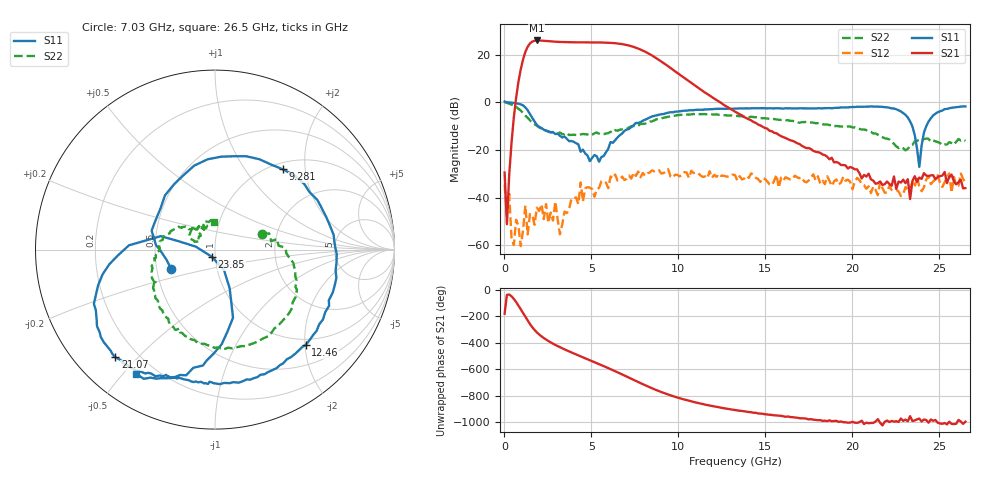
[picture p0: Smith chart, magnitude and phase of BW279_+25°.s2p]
!Agilent Technologies,N5242A,MY52422126,A.09.90.01
!Agilent N5242A: A.09.90.01
!Date: Thursday, November 28, 2013 10:13:04
!Correction: S11(Full 2 Port with power(1,2))
!S21(Full 2 Port with power(1,2))
!S12(Full 2 Port with power(1,2))
!S22(Full 2 Port with power(1,2))
!S2P File: Measurements: S11, S21, S12, S22:
# Hz S  RI  R 50
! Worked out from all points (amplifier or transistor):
!   201 points, 10 MHz to 26.5 GHz, reference 50 ohm
!   highest |S21| = 25.9 dB at 1.864 GHz (marker M1)
!   |S21| within 3 dB of that: 1.313 GHz to 7.542 GHz (6.229 GHz wide, 141 % of centre)
!   unconditionally stable (mu >= 1): 141 MHz to end of sweep
!   at 4.381 GHz: K = 1.46, MAG = 25.4 dB, |S12| = -33.7 dB
!   at 13.26 GHz: K = 9.21, MAG = 0.7 dB, |S12| = -30.6 dB
!   at 26.5 GHz: K = 499.98, MAG = -31.1 dB, |S12| = -33.8 dB
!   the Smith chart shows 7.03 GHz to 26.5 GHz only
!   S11 on the Smith chart (normalised r, x): 7.03 GHz: 0.59, -0.14; 9.281 GHz: 1.12, +1.53; 12.46 GHz: 0.88, -2.01; 21.07 GHz: 0.12, -0.43; 23.85 GHz: 0.96, -0.08; 26.5 GHz: 0.13, -0.54
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1e7  1.035 -0.0165  -0.0335 -0.000378  0.0178 0.00641  1.012 -0.0249
9.3715e8  -0.7386 -0.5224  -4.006 -2.793  -0.000378 -0.000878  -0.1887 -0.6407
1.20205e9  -0.7298 0.277  -10.49 4.382  -0.00671 0.00108  -0.3458 -0.3937
1.46695e9  -0.0688 0.5634  -3.729 16.79  -0.00419 0.00165  -0.3673 -0.2017
1.8643e9  0.3327 0.038  15.29 12.63  -0.00477 0.00386  -0.3187 -0.0149
2.26165e9  0.1501 -0.2196  19.51 -1.175  -0.000451 0.0035  -0.2439 0.0861
3.05635e9  -0.1626 -0.1472  8.103 -16.68  -0.00162 -0.00314  -0.1092 0.1919
3.7186e9  -0.1525 -0.00454  -4.622 -17.58  0.000565 0.00572  -0.00153 0.2057
4.5133e9  -0.0619 0.0804  -15.56 -9.176  0.000188 0.0083  0.095 0.1939
5.5729e9  0.0691 -0.0154  -15.8 8.585  0.0132 0.0174  0.1702 0.1282
6.3676e9  -0.0456 -0.1548  -4.573 16.75  0.0255 0.0167  0.225 0.1285
7.02985e9  -0.2447 -0.1077  6.749 14.39  0.0228 0.00913  0.2607 0.0894
7.82455e9  -0.3016 0.2351  12.33 3.291  0.0267 0.00286  0.3473 0.0583
8.88415e9  0.1743 0.5201  5.4 -5.531  0.0262 -0.0269  0.4402 -0.0946
9.2815e9  0.3786 0.4469  2.584 -5.601  0.0254 -0.0239  0.4543 -0.1718
1.24603e10  0.5048 -0.5318  -0.9571 -0.1526  -0.00488 -0.0281  -0.00252 -0.5475
1.3255e10  0.3794 -0.6341  -0.628 0.0939  -0.0157 -0.025  -0.1153 -0.5032
1.77583e10  -0.1869 -0.7184  -0.0135 0.0944  -0.0305 0.00428  -0.3522 -0.1222
2.106955e10  -0.5559 -0.5995  0.00674 0.0232  -0.00701 0.0103  -0.203 0.1271
2.212915e10  -0.659 -0.3923  0.00326 0.019  -0.00874 0.0152  -0.1167 0.1175
2.3851e10  -0.0164 -0.0409  -0.00757 0.0252  -0.00722 0.0149  -0.1419 0.0798
2.65e10  -0.4376 -0.6923  0.00192 0.0156  0.00745 0.019  -0.00759 0.1547
